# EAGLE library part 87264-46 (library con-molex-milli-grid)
RECEPTACAL
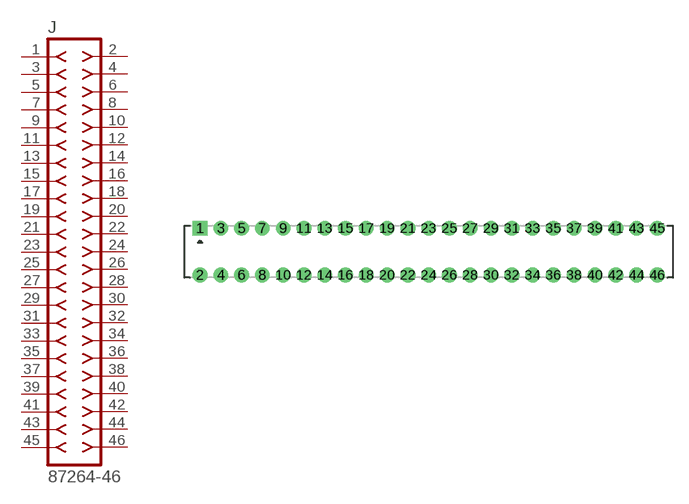
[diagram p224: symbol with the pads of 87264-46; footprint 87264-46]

Designator prefix J

## 87264-46  [87264-46]
1  1  pas
2  2  pas
3  3  pas
4  4  pas
5  5  pas
6  6  pas
7  7  pas
8  8  pas
9  9  pas
10  10  pas
11  11  pas
12  12  pas
13  13  pas
14  14  pas
15  15  pas
16  16  pas
17  17  pas
18  18  pas
19  19  pas
20  20  pas
21  21  pas
22  22  pas
23  23  pas
24  24  pas
25  25  pas
26  26  pas
27  27  pas
28  28  pas
29  29  pas
30  30  pas
31  31  pas
32  32  pas
33  33  pas
34  34  pas
35  35  pas
36  36  pas
37  37  pas
38  38  pas
39  39  pas
40  40  pas
41  41  pas
42  42  pas
43  43  pas
44  44  pas
45  45  pas
46  46  pas

## Footprint 87264-46 (pad centres in mm)
RECEPTACAL Dual Row, Side Entry
drill 0.914 square: 1 -22,2.25
drill 0.914: 2 -22,-2.25; 3 -20,2.25; 4 -20,-2.25; 5 -18,2.25; 6 -18,-2.25; 7 -16,2.25; 8 -16,-2.25; 9 -14,2.25; 10 -14,-2.25; 11 -12,2.25; 12 -12,-2.25; 13 -10,2.25; 14 -10,-2.25; 15 -8,2.25; 16 -8,-2.25; 17 -6,2.25; 18 -6,-2.25; 19 -4,2.25; 20 -4,-2.25; 21 -2,2.25; 22 -2,-2.25; 23 0,2.25; 24 0,-2.25; 25 2,2.25; 26 2,-2.25; 27 4,2.25; 28 4,-2.25; 29 6,2.25; 30 6,-2.25; 31 8,2.25; 32 8,-2.25; 33 10,2.25; 34 10,-2.25; 35 12,2.25; 36 12,-2.25; 37 14,2.25; 38 14,-2.25; 39 16,2.25; 40 16,-2.25; 41 18,2.25; 42 18,-2.25; 43 20,2.25; 44 20,-2.25; 45 22,2.25; 46 22,-2.25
